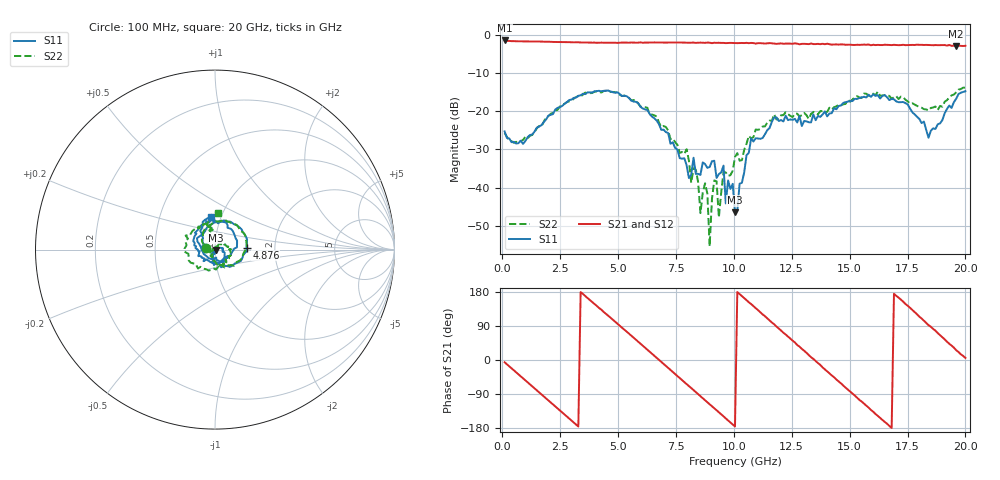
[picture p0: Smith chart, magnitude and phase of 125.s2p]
!Agilent Technologies,N5230C,MY49001569,A.09.33.09
!Agilent N5230C: A.09.33.09
!Date: Monday, July 27, 2015 15:31:42
!Correction: S11(Full 2 Port(1,2))
!S21(Full 2 Port(1,2))
!S12(Full 2 Port(1,2))
!S22(Full 2 Port(1,2))
!S2P File: Measurements: S11, S21, S12, S22:
# Hz S  dB  R 50
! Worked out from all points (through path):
!   201 points, 100 MHz to 20 GHz, reference 50 ohm
!   highest |S21| = -1.40 dB at 100 MHz (marker M1); lowest = -2.9 dB at 19.6 GHz (marker M2)
!   group delay of S21, straight-line fit = 149 ps
!   lowest |S11| = -46.5 dB at 10.05 GHz (marker M3), VSWR 1.01, Z = 50.4 - j0.222 ohm
!   |S11| at or under -10 dB: start of sweep to end of sweep
!   |S22| runs from -55.4 to -13.8 dB; largest |S21 - S12| = 0.033
!   S11 on the Smith chart (normalised r, x): 100 MHz: 0.90, +0.02; 4.876 GHz: 1.43, +0.03; 20 GHz: 0.90, +0.34
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1e8  -25.27 169.3  -1.40 -6.0  -1.44 -6.0  -25.73 169.6
1.692e9  -23.62 155.3  -1.70 -91.2  -1.76 -91.1  -23.90 154.8
3.483e9  -15.38 72.6  -1.93 174.3  -1.95 174.0  -15.64 77.2
4.876e9  -15.08 3.6  -2.00 101.0  -2.00 101.3  -15.05 5.4
6.7665e9  -23.37 -90.9  -1.93 0.6  -1.93 0.5  -22.98 -87.3
7.9605e9  -34.16 -125.2  -1.98 -63.6  -1.97 -63.2  -29.95 -148.7
8.5575e9  -36.70 -63.9  -1.97 -95.6  -2.02 -95.2  -46.72 -143.6
8.7565e9  -33.86 -82.3  -2.03 -106.0  -2.00 -105.7  -38.88 138.8
8.9555e9  -34.62 -64.8  -1.99 -117.0  -1.98 -116.7  -55.40 -134.1
9.1545e9  -32.97 -104.5  -2.00 -127.3  -1.98 -127.2  -38.12 86.0
9.3535e9  -36.47 -79.3  -2.01 -137.8  -2.08 -138.0  -47.85 139.6
9.5525e9  -34.26 -115.8  -2.04 -148.5  -2.06 -148.5  -35.92 61.2
9.652e9  -44.18 -116.8  -2.10 -154.2  -2.03 -153.5  -36.06 81.7
1.005e10  -46.52 -27.8  -2.07 -175.5  -2.07 -175.3  -32.00 59.0
1.07465e10  -27.13 11.7  -2.05 147.6  -2.14 147.5  -27.11 41.2
1.1642e10  -22.75 -43.2  -2.14 99.0  -2.16 99.5  -22.49 12.1
1.3433e10  -20.81 -135.0  -2.35 2.9  -2.30 2.9  -20.14 -61.3
1.51245e10  -17.30 139.4  -2.57 -88.8  -2.39 -88.2  -16.91 -147.2
1.67165e10  -17.04 60.3  -2.58 -174.0  -2.59 -173.7  -15.96 130.7
1.83085e10  -24.89 -82.7  -2.56 97.8  -2.61 99.6  -19.50 100.5
1.9602e10  -16.71 118.2  -2.88 25.8  -2.65 27.9  -15.04 97.2
2e10  -14.73 96.7  -2.81 5.5  -2.94 4.5  -13.80 85.9
